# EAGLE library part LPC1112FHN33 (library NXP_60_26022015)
32-bit ARM Cortex-M0 microcontroller; up to 64 kB flash and 8 kB SRAM The LPC1110/11/12/13/14/15 are a ARM Cortex-M0 based, low-cost 32-bit MCU family, designed for 8/16-bit microcontroller applications, offering performance, low power, simple instruction set and memory addressing together with reduced code size compared to existing 8/16-bit architectures. The LPC1110/11/12/13/14/15 operate at CPU frequencies of up to 50 MHz. The peripheral complement of the LPC1110/11/12/13/14/15 includes up to 64 kB of flash memory, up to 8 kB of data memory, one Fast-mode Plus I 2 C-bus interface, one RS-485/EIA-485 UART, up to two SPI interfaces with SSP features, four general purpose counter/timers, a 10-bit ADC, and up to 42 general purpose I/O pins. Remark: The LPC111x series consists of the LPC1100 series (parts LPC111x/101/201/301), LPC1100L series (parts LPC111x/002/102/202/302), and the LPC1100XL series (parts LPC111x/103/203/303/323/333). The LPC1100L and LPC1100XL series include the power profiles, a windowed watchdog timer, and a configurable open-drain mode. AAL Eindhoven MK
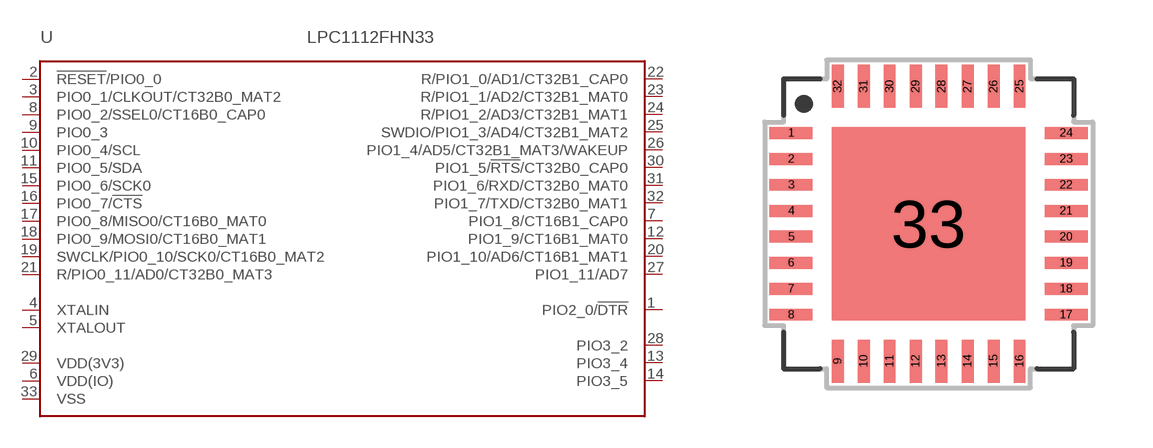
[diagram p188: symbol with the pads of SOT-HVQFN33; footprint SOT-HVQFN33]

Designator prefix U

## LPC1112FHN33/101 (ADC: 8; FLASH: 16kB; GPIO: 28; PWR_PROFILES: no; SERIES: LPC1100; SPI: 1; SRAM: 2kB), LPC1112FHN33/102 (ADC: 8; FLASH: 16kB; GPIO: 28; PWR_PROFILES: yes; SERIES: LPC1100L; SPI: 1; SRAM: 2kB), LPC1112FHN33/201 (ADC: 8; FLASH: 16kB; GPIO: 28; PWR_PROFILES: no; SERIES: LPC1100; SPI: 1; SRAM: 4kB), LPC1112FHN33/202 (ADC: 8; FLASH: 16KB; GPIO: 28; PWR_PROFILES: yes; SERIES: LPC1100L; SPI: 1; SRAM: 4kB)  [SOT-HVQFN33]
1  PIO2_0/!DTR!
2  !RESET!/PIO0_0
3  PIO0_1/CLKOUT/CT32B0_MAT2
4  XTALIN  in
5  XTALOUT  out
6  VDD(IO)  pwr
7  PIO1_8/CT16B1_CAP0
8  PIO0_2/SSEL0/CT16B0_CAP0
9  PIO0_3
10  PIO0_4/SCL
11  PIO0_5/SDA
12  PIO1_9/CT16B1_MAT0
13  PIO3_4
14  PIO3_5
15  PIO0_6/SCK0
16  PIO0_7/!CTS!
17  PIO0_8/MISO0/CT16B0_MAT0
18  PIO0_9/MOSI0/CT16B0_MAT1
19  SWCLK/PIO0_10/SCK0/CT16B0_MAT2
20  PIO1_10/AD6/CT16B1_MAT1
21  R/PIO0_11/AD0/CT32B0_MAT3
22  R/PIO1_0/AD1/CT32B1_CAP0
23  R/PIO1_1/AD2/CT32B1_MAT0
24  R/PIO1_2/AD3/CT32B1_MAT1
25  SWDIO/PIO1_3/AD4/CT32B1_MAT2
26  PIO1_4/AD5/CT32B1_MAT3/WAKEUP
27  PIO1_11/AD7
28  PIO3_2
29  VDD(3V3)  pwr
30  PIO1_5/!RTS!/CT32B0_CAP0
31  PIO1_6/RXD/CT32B0_MAT0
32  PIO1_7/TXD/CT32B0_MAT1
33  VSS  pwr

## Footprint SOT-HVQFN33 (pad centres in mm)
SOTxxx HVQFN33: plastic thermal enhanced very thin quad flat package; no leads; 33 terminals; body 7 x 7 x 0.85 mm JEDEC: --- IEC: --- Package according LPC111x datasheet
smd 1.075 x 0.3: 1 -3.438,2.275; 2 -3.438,1.625; 3 -3.438,0.975; 4 -3.438,0.325; 5 -3.438,-0.325; 6 -3.438,-0.975; 7 -3.438,-1.625; 8 -3.438,-2.275; 17 3.438,-2.275; 18 3.438,-1.625; 19 3.438,-0.975; 20 3.438,-0.325; 21 3.438,0.325; 22 3.438,0.975; 23 3.438,1.625; 24 3.438,2.275
smd 0.3 x 1.075: 9 -2.275,-3.438; 10 -1.625,-3.438; 11 -0.975,-3.438; 12 -0.325,-3.438; 13 0.325,-3.438; 14 0.975,-3.438; 15 1.625,-3.438; 16 2.275,-3.438; 25 2.275,3.438; 26 1.625,3.438; 27 0.975,3.438; 28 0.325,3.438; 29 -0.325,3.438; 30 -0.975,3.438; 31 -1.625,3.438; 32 -2.275,3.438
smd 4.85 x 4.85: 33 0,0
